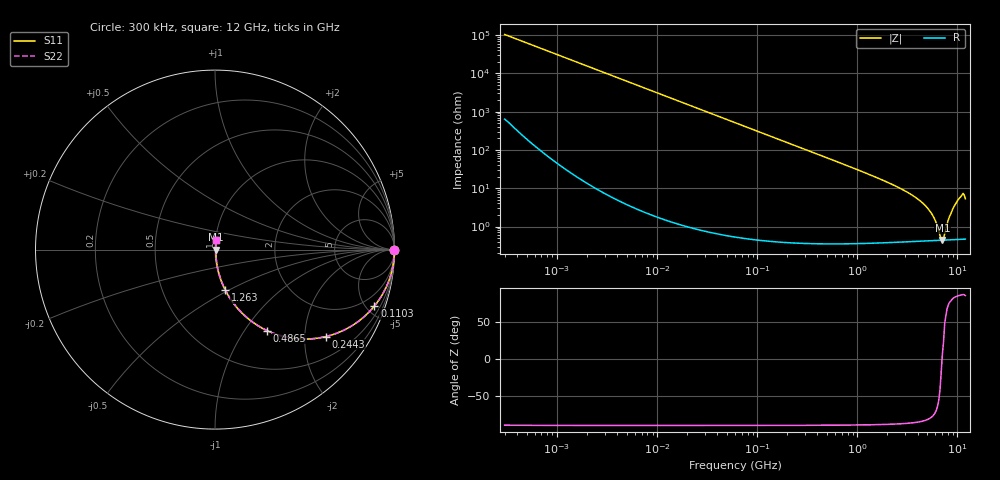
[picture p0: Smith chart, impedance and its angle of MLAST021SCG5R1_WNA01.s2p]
! MLAST021SCG5R1_WNA01  S-PARAMETER MODEL  ( General Type )
! Model Generated by TAIYO YUDEN Corporation (http://www.ty-top.com)
! Version 1.0
! TAIYO YUDEN Control No. 220901
! Copyright(c) 2022 TAIYO YUDEN CO.,LTD. All Rights Reserved.
! Product Description (link to TY-COMPAS)
! https://ds.yuden.co.jp/TYCOMPAS/or/detail?pn=MLAST021SCG5R1CWNA01&u=M
! Products Name : Multilayer Ceramic Capacitors
! Characteristics :
!  Capacitance : 5.1 pF , Rated Voltage : 25V , TCC : CG / C0G
!  Case Size : 0.25 x 0.125 / 0.0098 x 0.0049 [mm/inch] , Thickness : 0.125 / 0.0049 [mm/inch]
!  (Conditions: Temperature = 25 degC , DC Bias Current/Voltage = 0A / 0V)
! External Node Assignments :
!  1  o---| |---o  2
! GND o---------o GND
! Frequency Range : 0.3MHz  -  12000MHz  [ 401 STEP ]
# MHz S RI R 50
! Freq[MHz].  S11 Real  S11 Imag  S21 Real  S21 Imag  S12 Real  S12 Imag  S22 Real  S22 Imag
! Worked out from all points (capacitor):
!   401 points, 300 kHz to 12 GHz, reference 50 ohm
!   read as one part in series: C = 5.1 pF near 316.3 kHz
!   lowest |Z| = 443 mohm at 7.064 GHz (marker M1)
!   series resonance near 7.025 GHz, so ESL is about 100 pH
!   S11 on the Smith chart (normalised r, x): 300 kHz: open; 110.3 MHz: 1.01, -5.65; 244.3 MHz: 1.01, -2.55; 486.5 MHz: 1.01, -1.28; 1.263 GHz: 1.01, -0.48; 12 GHz: 1.01, +0.11
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0.3  1 -0.000961  6.84e-06 0.000961  6.84e-06 0.000961  1 -0.000961
1.769972  1 -0.00567  3.74e-05 0.00567  3.74e-05 0.00567  1 -0.00567
10.44266  0.9989 -0.0334  0.00114 0.0334  0.00114 0.0334  0.9989 -0.0334
60  0.9642 -0.1854  0.0358 0.1854  0.0358 0.1854  0.9642 -0.1854
110.3493  0.8884 -0.3141  0.1116 0.3141  0.1116 0.3141  0.8884 -0.3141
244.3004  0.6191 -0.4842  0.3809 0.4842  0.3809 0.4842  0.6191 -0.4842
353.9943  0.4363 -0.4939  0.5637 0.4939  0.5637 0.4939  0.4363 -0.4939
486.4723  0.2906 -0.4513  0.7094 0.4513  0.7094 0.4513  0.2906 -0.4513
763.2128  0.1425 -0.3452  0.8575 0.3452  0.8575 0.3452  0.1425 -0.3452
1262.535  0.0571 -0.2246  0.9429 0.2246  0.9429 0.2246  0.0571 -0.2246
2088.533  0.0218 -0.1326  0.9782 0.1326  0.9782 0.1326  0.0218 -0.1326
3454.93  0.00861 -0.0674  0.9914 0.0674  0.9914 0.0674  0.00861 -0.0674
4747.894  0.00542 -0.0351  0.9946 0.0351  0.9946 0.0351  0.00542 -0.0351
5715.274  0.00461 -0.018  0.9954 0.018  0.9954 0.018  0.00461 -0.018
6188.031  0.00444 -0.0109  0.9956 0.0109  0.9956 0.0109  0.00444 -0.0109
6699.894  0.00438 -0.00382  0.9956 0.00382  0.9956 0.00382  0.00438 -0.00382
7064.448  0.00439 0.000397  0.9956 -0.000397  0.9956 -0.000397  0.00439 0.000397
7448.838  0.00444 0.00465  0.9956 -0.00465  0.9956 -0.00465  0.00444 0.00465
8503.825  0.00488 0.0196  0.9951 -0.0196  0.9951 -0.0196  0.00488 0.0196
9454.42  0.00588 0.0364  0.9941 -0.0364  0.9941 -0.0364  0.00588 0.0364
10793.46  0.00816 0.0593  0.9918 -0.0593  0.9918 -0.0593  0.00816 0.0593
12000  0.00744 0.0525  0.9926 -0.0525  0.9926 -0.0525  0.00744 0.0525
